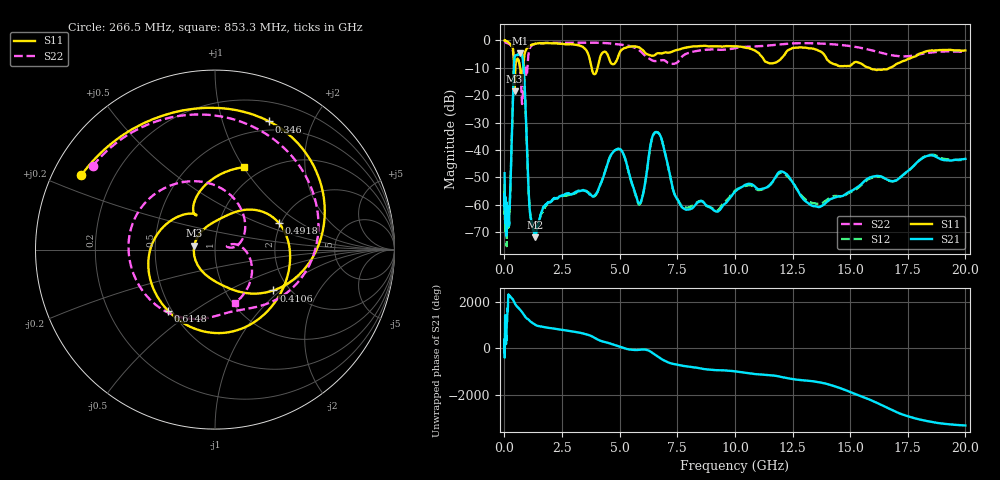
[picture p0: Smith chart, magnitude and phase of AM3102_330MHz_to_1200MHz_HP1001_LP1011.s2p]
! Date/Time: Tue, Sep 11, 2018 5:18 PM
! Network Analyzer: Agilent Technologies E8362B Rev: A.07.50.63
! Sweep from 0.010 to 20.000 GHz, 1601 Points, Sweep Type: LOG
! Power Supply: 4.949 V, 0.001 A
# Hz S DB R 50
!freq MagS11 AngS11 MagS21 AngS21 MagS12 AngS12 MagS22 AngS22
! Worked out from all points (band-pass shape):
!   1601 points, 10 MHz to 20 GHz, reference 50 ohm
!   highest |S21| = -4.69 dB at 695.6 MHz (marker M1); lowest = -71.9 dB at 1.321 GHz (marker M2)
!   |S21| within 3 dB of the highest: 425.9 MHz to 808.9 MHz (383.1 MHz wide, 62 % of centre)
!   lowest |S11| = -18.6 dB at 443 MHz (marker M3), VSWR 1.27, Z = 39.6 + j1.73 ohm
!   |S11| at or under -10 dB: 684.4 MHz to 812.4 MHz (128 MHz wide, 17.1 % of centre); 3.787 GHz to 4.043 GHz (256 MHz wide, 6.54 % of centre); 15.84 GHz to 16.72 GHz (886.7 MHz wide, 5.45 % of centre)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
!   |S22| runs from -23.2 to -0.2 dB; largest |S21 - S12| = 0.01
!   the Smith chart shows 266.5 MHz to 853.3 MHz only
!   S11 on the Smith chart (normalised r, x): 266.5 MHz: 0.09, +0.26; 346 MHz: 0.40, +1.43; 410.6 MHz: 1.66, -0.90; 491.8 MHz: 1.94, +0.68; 614.8 MHz: 0.48, -0.40; 853.3 MHz: 0.84, +1.01
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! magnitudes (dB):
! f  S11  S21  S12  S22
! 10 MHz  0.0  -48.5  -52.3  -0.2
! 35.55 MHz  0.0  -64.1  -65.1  -0.5
! 126.4 MHz  -0.4  -65.2  -63.5  -1.0
! 266.5 MHz  -1.4  -52.5  -52.4  -1.7
! 346 MHz  -2.2  -28.2  -28.3  -2.9
! 410.6 MHz  -8.0  -10.2  -10.2  -6.5
! 443 MHz  -18.6  -6.2  -6.2  -8.9
! 447.2 MHz  -18.4  -6.0  -6.0  -8.9
! 491.8 MHz  -8.3  -5.4  -5.4  -7.2
! 614.8 MHz  -7.3  -4.9  -5.1  -7.2
! 695.6 MHz  -10.7  -4.7  -4.7  -11.8
! 772.3 MHz  -13.0  -5.7  -5.7  -23.2
! 853.3 MHz  -6.2  -12.6  -12.7  -10.0
! 1.087 GHz  -2.0  -60.3  -60.5  -3.3
! 1.321 GHz  -1.2  -71.9  -71.4  -1.3
! 1.59 GHz  -1.0  -63.2  -63.4  -1.0
! 3.921 GHz  -12.3  -56.5  -56.8  -0.8
! 4.902 GHz  -6.7  -39.6  -39.7  -1.4
! 5.652 GHz  -2.2  -55.1  -55.7  -2.6
! 6.612 GHz  -4.8  -33.5  -33.5  -7.5
! 7.92 GHz  -2.5  -61.8  -61.1  -4.8
! 20 GHz  -3.6  -43.3  -43.8  -4.1
